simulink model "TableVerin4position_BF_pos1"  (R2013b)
settings: Solver=ode15s  StartTime=0.0  StopTime=10  RelTol=1e-3
undefined symbols (not defined in the file): deg, kg, m, mm, N, rad, s, X, Y, Z
libraries: sm_lib x907, fl_lib x24, nesl_utility x18, elec_lib x3, sdl_lib x2, simulink x1
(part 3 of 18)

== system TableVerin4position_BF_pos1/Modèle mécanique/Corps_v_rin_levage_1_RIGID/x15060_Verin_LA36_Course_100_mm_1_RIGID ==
  ReferenceFrame : sm_lib/Frames and Transforms/Reference Frame  BlockFunction=simmechanics.library.frames_transforms.reference_frame
  Solid : sm_lib/Body Elements/Solid  InertiaType=Custom  Mass=16.4344  MassUnits=kg  CenterOfMass=[-32.3232 0.0025488500000000001 17.760100000000001]  CenterOfMassUnits=mm  MomentsOfInertia=[90976.899999999994 107643 28123.599999999999]  MomentsOfInertiaUnits=kg*mm^2  ProductsOfInertia=[5.1204799999999997 -235.90300000000005 -1.9517]  ProductsOfInertiaUnits=kg*mm^2  DensityBased=on  Density=1000  DensityUnits=kg/(m^3)  GraphicType=FromGeometry  MarkerShape=Sphere  MarkerSize=10  MarkerSizeUnits=m  GraphicVisPropType=SimpleVisualProperties  GraphicDiffuseColor=[0.647059 0.517647 0]  GraphicSpecularColor=[0.5 0.5 0.5 1.0]  GraphicAmbientColor=[0.15 0.15 0.15 1.0]  GraphicEmissiveColor=[0.0 0.0 0.0 1.0]  GraphicShininess=75  GraphicOpacity=1  GeometryShape=FromFile  RectangleSize=[1 1]  RectangleSizeUnits=m  BrickDimensions=[1 1 1]  BrickDimensionUnits=m  CylinderRadius=1  CylinderRadiusUnits=m  CylinderLength=1  CylinderLengthUnits=m  SphereRadius=1  SphereRadiusUnits=m  EllipsoidRadii=[1 1 1]  EllipsoidRadiiUnits=m  ExtrusionCrossSection=[1 1; -1 1; -1 -1; 1 -1]  ExtrusionCrossSectionUnits=m  ExtrusionLength=1  ExtrusionLengthUnits=m  PolygonNumSides=3  PolygonOuterRadius=1  PolygonOuterRadiusUnits=m  ExtGeomFileName=15060-Verin - LA36 - Course 100 mm_Défaut_sldprt.STL  ExtGeomFileUnits=mm  RevolutionCrossSection=[1 1; 1 -1; 2 -1; 2 1]  RevolutionCrossSectionUnits=m  RevolutionExtent=Full  RevolutionAngle=180  RevolutionAngleUnits=deg  BlockFunction=simmechanics.library.body_elements.solid
  F : PMIOPort  Port=1  Side=Left
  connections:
  Solid/RConn1 -- ReferenceFrame/RConn1 -- F/RConn1

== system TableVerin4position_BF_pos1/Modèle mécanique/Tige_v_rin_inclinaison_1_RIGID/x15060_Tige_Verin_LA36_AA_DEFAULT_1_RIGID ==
  ReferenceFrame : sm_lib/Frames and Transforms/Reference Frame  BlockFunction=simmechanics.library.frames_transforms.reference_frame
  Solid : sm_lib/Body Elements/Solid  InertiaType=Custom  Mass=1.0865400000000001  MassUnits=kg  CenterOfMass=[100.095 0 0]  CenterOfMassUnits=mm  MomentsOfInertia=[122.032 3676.6300000000001 3676.6300000000001]  MomentsOfInertiaUnits=kg*mm^2  ProductsOfInertia=[0 0 0]  ProductsOfInertiaUnits=kg*mm^2  DensityBased=on  Density=1000  DensityUnits=kg/(m^3)  GraphicType=FromGeometry  MarkerShape=Sphere  MarkerSize=10  MarkerSizeUnits=m  GraphicVisPropType=SimpleVisualProperties  GraphicDiffuseColor=[0.776471 0.756863 0.737255]  GraphicSpecularColor=[0.5 0.5 0.5 1.0]  GraphicAmbientColor=[0.15 0.15 0.15 1.0]  GraphicEmissiveColor=[0.0 0.0 0.0 1.0]  GraphicShininess=75  GraphicOpacity=1  GeometryShape=FromFile  RectangleSize=[1 1]  RectangleSizeUnits=m  BrickDimensions=[1 1 1]  BrickDimensionUnits=m  CylinderRadius=1  CylinderRadiusUnits=m  CylinderLength=1  CylinderLengthUnits=m  SphereRadius=1  SphereRadiusUnits=m  EllipsoidRadii=[1 1 1]  EllipsoidRadiiUnits=m  ExtrusionCrossSection=[1 1; -1 1; -1 -1; 1 -1]  ExtrusionCrossSectionUnits=m  ExtrusionLength=1  ExtrusionLengthUnits=m  PolygonNumSides=3  PolygonOuterRadius=1  PolygonOuterRadiusUnits=m  ExtGeomFileName=15060-Tige Verin - LA36_AA - DEFAULT_Défaut_sldprt.STL  ExtGeomFileUnits=mm  RevolutionCrossSection=[1 1; 1 -1; 2 -1; 2 1]  RevolutionCrossSectionUnits=m  RevolutionExtent=Full  RevolutionAngle=180  RevolutionAngleUnits=deg  BlockFunction=simmechanics.library.body_elements.solid
  F : PMIOPort  Port=1  Side=Left
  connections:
  Solid/RConn1 -- ReferenceFrame/RConn1 -- F/RConn1

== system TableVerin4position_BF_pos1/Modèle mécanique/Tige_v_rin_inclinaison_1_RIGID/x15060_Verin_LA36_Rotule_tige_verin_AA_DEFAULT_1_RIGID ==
  ReferenceFrame : sm_lib/Frames and Transforms/Reference Frame  BlockFunction=simmechanics.library.frames_transforms.reference_frame
  Solid : sm_lib/Body Elements/Solid  InertiaType=Custom  Mass=0.218778  MassUnits=kg  CenterOfMass=[17.366699999999998 -1.65342e-06 4.7137100000000001e-06]  CenterOfMassUnits=mm  MomentsOfInertia=[24.659199999999998 72.896000000000001 84.362000000000009]  MomentsOfInertiaUnits=kg*mm^2  ProductsOfInertia=[-4.0241599999999998e-05 3.5702500000000002e-06 -2.8363700000000001e-06]  ProductsOfInertiaUnits=kg*mm^2  DensityBased=on  Density=1000  DensityUnits=kg/(m^3)  GraphicType=FromGeometry  MarkerShape=Sphere  MarkerSize=10  MarkerSizeUnits=m  GraphicVisPropType=SimpleVisualProperties  GraphicDiffuseColor=[0.776471 0.756863 0.737255]  GraphicSpecularColor=[0.5 0.5 0.5 1.0]  GraphicAmbientColor=[0.15 0.15 0.15 1.0]  GraphicEmissiveColor=[0.0 0.0 0.0 1.0]  GraphicShininess=75  GraphicOpacity=1  GeometryShape=FromFile  RectangleSize=[1 1]  RectangleSizeUnits=m  BrickDimensions=[1 1 1]  BrickDimensionUnits=m  CylinderRadius=1  CylinderRadiusUnits=m  CylinderLength=1  CylinderLengthUnits=m  SphereRadius=1  SphereRadiusUnits=m  EllipsoidRadii=[1 1 1]  EllipsoidRadiiUnits=m  ExtrusionCrossSection=[1 1; -1 1; -1 -1; 1 -1]  ExtrusionCrossSectionUnits=m  ExtrusionLength=1  ExtrusionLengthUnits=m  PolygonNumSides=3  PolygonOuterRadius=1  PolygonOuterRadiusUnits=m  ExtGeomFileName=15060-Verin - LA36 - Rotule tige verin_AA - DEFAULT_Défaut_sldprt.STL  ExtGeomFileUnits=mm  RevolutionCrossSection=[1 1; 1 -1; 2 -1; 2 1]  RevolutionCrossSectionUnits=m  RevolutionExtent=Full  RevolutionAngle=180  RevolutionAngleUnits=deg  BlockFunction=simmechanics.library.body_elements.solid
  F : PMIOPort  Port=1  Side=Left
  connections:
  Solid/RConn1 -- ReferenceFrame/RConn1 -- F/RConn1

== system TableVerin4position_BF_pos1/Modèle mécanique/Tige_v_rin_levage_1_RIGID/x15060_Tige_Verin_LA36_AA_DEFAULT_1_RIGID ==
  ReferenceFrame : sm_lib/Frames and Transforms/Reference Frame  BlockFunction=simmechanics.library.frames_transforms.reference_frame
  Solid : sm_lib/Body Elements/Solid  InertiaType=Custom  Mass=1.0865400000000001  MassUnits=kg  CenterOfMass=[100.095 0 0]  CenterOfMassUnits=mm  MomentsOfInertia=[122.032 3676.6300000000001 3676.6300000000001]  MomentsOfInertiaUnits=kg*mm^2  ProductsOfInertia=[0 0 0]  ProductsOfInertiaUnits=kg*mm^2  DensityBased=on  Density=1000  DensityUnits=kg/(m^3)  GraphicType=FromGeometry  MarkerShape=Sphere  MarkerSize=10  MarkerSizeUnits=m  GraphicVisPropType=SimpleVisualProperties  GraphicDiffuseColor=[0.776471 0.756863 0.737255]  GraphicSpecularColor=[0.5 0.5 0.5 1.0]  GraphicAmbientColor=[0.15 0.15 0.15 1.0]  GraphicEmissiveColor=[0.0 0.0 0.0 1.0]  GraphicShininess=75  GraphicOpacity=1  GeometryShape=FromFile  RectangleSize=[1 1]  RectangleSizeUnits=m  BrickDimensions=[1 1 1]  BrickDimensionUnits=m  CylinderRadius=1  CylinderRadiusUnits=m  CylinderLength=1  CylinderLengthUnits=m  SphereRadius=1  SphereRadiusUnits=m  EllipsoidRadii=[1 1 1]  EllipsoidRadiiUnits=m  ExtrusionCrossSection=[1 1; -1 1; -1 -1; 1 -1]  ExtrusionCrossSectionUnits=m  ExtrusionLength=1  ExtrusionLengthUnits=m  PolygonNumSides=3  PolygonOuterRadius=1  PolygonOuterRadiusUnits=m  ExtGeomFileName=15060-Tige Verin - LA36_AA - DEFAULT_Défaut_sldprt.STL  ExtGeomFileUnits=mm  RevolutionCrossSection=[1 1; 1 -1; 2 -1; 2 1]  RevolutionCrossSectionUnits=m  RevolutionExtent=Full  RevolutionAngle=180  RevolutionAngleUnits=deg  BlockFunction=simmechanics.library.body_elements.solid
  F : PMIOPort  Port=1  Side=Left
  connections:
  Solid/RConn1 -- ReferenceFrame/RConn1 -- F/RConn1

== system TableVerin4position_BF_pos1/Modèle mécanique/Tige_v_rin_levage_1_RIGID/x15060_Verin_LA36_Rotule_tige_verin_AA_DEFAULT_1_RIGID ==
  ReferenceFrame : sm_lib/Frames and Transforms/Reference Frame  BlockFunction=simmechanics.library.frames_transforms.reference_frame
  Solid : sm_lib/Body Elements/Solid  InertiaType=Custom  Mass=0.218778  MassUnits=kg  CenterOfMass=[17.366699999999998 -1.65342e-06 4.7137100000000001e-06]  CenterOfMassUnits=mm  MomentsOfInertia=[24.659199999999998 72.896000000000001 84.362000000000009]  MomentsOfInertiaUnits=kg*mm^2  ProductsOfInertia=[-4.0241599999999998e-05 3.5702500000000002e-06 -2.8363700000000001e-06]  ProductsOfInertiaUnits=kg*mm^2  DensityBased=on  Density=1000  DensityUnits=kg/(m^3)  GraphicType=FromGeometry  MarkerShape=Sphere  MarkerSize=10  MarkerSizeUnits=m  GraphicVisPropType=SimpleVisualProperties  GraphicDiffuseColor=[0.776471 0.756863 0.737255]  GraphicSpecularColor=[0.5 0.5 0.5 1.0]  GraphicAmbientColor=[0.15 0.15 0.15 1.0]  GraphicEmissiveColor=[0.0 0.0 0.0 1.0]  GraphicShininess=75  GraphicOpacity=1  GeometryShape=FromFile  RectangleSize=[1 1]  RectangleSizeUnits=m  BrickDimensions=[1 1 1]  BrickDimensionUnits=m  CylinderRadius=1  CylinderRadiusUnits=m  CylinderLength=1  CylinderLengthUnits=m  SphereRadius=1  SphereRadiusUnits=m  EllipsoidRadii=[1 1 1]  EllipsoidRadiiUnits=m  ExtrusionCrossSection=[1 1; -1 1; -1 -1; 1 -1]  ExtrusionCrossSectionUnits=m  ExtrusionLength=1  ExtrusionLengthUnits=m  PolygonNumSides=3  PolygonOuterRadius=1  PolygonOuterRadiusUnits=m  ExtGeomFileName=15060-Verin - LA36 - Rotule tige verin_AA - DEFAULT_Défaut_sldprt.STL  ExtGeomFileUnits=mm  RevolutionCrossSection=[1 1; 1 -1; 2 -1; 2 1]  RevolutionCrossSectionUnits=m  RevolutionExtent=Full  RevolutionAngle=180  RevolutionAngleUnits=deg  BlockFunction=simmechanics.library.body_elements.solid
  F : PMIOPort  Port=1  Side=Left
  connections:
  Solid/RConn1 -- ReferenceFrame/RConn1 -- F/RConn1

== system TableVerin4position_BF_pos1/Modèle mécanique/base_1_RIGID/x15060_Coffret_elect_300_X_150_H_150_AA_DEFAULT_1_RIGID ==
  ReferenceFrame : sm_lib/Frames and Transforms/Reference Frame  BlockFunction=simmechanics.library.frames_transforms.reference_frame
  Solid : sm_lib/Body Elements/Solid  InertiaType=Custom  Mass=0.83252499999999996  MassUnits=kg  CenterOfMass=[0 0 86.964399999999998]  CenterOfMassUnits=mm  MomentsOfInertia=[9125.25 3583.1799999999998 10424.799999999999]  MomentsOfInertiaUnits=kg*mm^2  ProductsOfInertia=[0 0 0]  ProductsOfInertiaUnits=kg*mm^2  DensityBased=on  Density=1000  DensityUnits=kg/(m^3)  GraphicType=FromGeometry  MarkerShape=Sphere  MarkerSize=10  MarkerSizeUnits=m  GraphicVisPropType=SimpleVisualProperties  GraphicDiffuseColor=[0.792157 0.819608 0.933333]  GraphicSpecularColor=[0.5 0.5 0.5 1.0]  GraphicAmbientColor=[0.15 0.15 0.15 1.0]  GraphicEmissiveColor=[0.0 0.0 0.0 1.0]  GraphicShininess=75  GraphicOpacity=1  GeometryShape=FromFile  RectangleSize=[1 1]  RectangleSizeUnits=m  BrickDimensions=[1 1 1]  BrickDimensionUnits=m  CylinderRadius=1  CylinderRadiusUnits=m  CylinderLength=1  CylinderLengthUnits=m  SphereRadius=1  SphereRadiusUnits=m  EllipsoidRadii=[1 1 1]  EllipsoidRadiiUnits=m  ExtrusionCrossSection=[1 1; -1 1; -1 -1; 1 -1]  ExtrusionCrossSectionUnits=m  ExtrusionLength=1  ExtrusionLengthUnits=m  PolygonNumSides=3  PolygonOuterRadius=1  PolygonOuterRadiusUnits=m  ExtGeomFileName=15060-Coffret elect - 300 X 150 H 150_AA - DEFAULT_Défaut_sldprt.STL  ExtGeomFileUnits=mm  RevolutionCrossSection=[1 1; 1 -1; 2 -1; 2 1]  RevolutionCrossSectionUnits=m  RevolutionExtent=Full  RevolutionAngle=180  RevolutionAngleUnits=deg  BlockFunction=simmechanics.library.body_elements.solid
  F : PMIOPort  Port=1  Side=Left
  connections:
  Solid/RConn1 -- ReferenceFrame/RConn1 -- F/RConn1

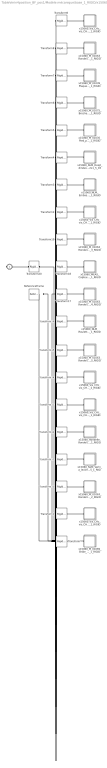
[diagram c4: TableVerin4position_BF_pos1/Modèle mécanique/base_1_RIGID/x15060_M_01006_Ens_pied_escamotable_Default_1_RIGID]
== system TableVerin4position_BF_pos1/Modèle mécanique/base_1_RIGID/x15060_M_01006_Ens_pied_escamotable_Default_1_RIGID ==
  ReferenceFrame : sm_lib/Frames and Transforms/Reference Frame  BlockFunction=simmechanics.library.frames_transforms.reference_frame
  Transform : sm_lib/Frames and Transforms/Rigid Transform  TranslationMethod=Cartesian  TranslationLengthUnit=mm  TranslationStandardAxis=+Z  TranslationStandardOffset=0  TranslationCartesianOffset=[-28 52.5 1]  TranslationROffset=0  TranslationROffsetUnits=m  TranslationZOffset=0  TranslationZOffsetUnits=m  TranslationThetaOffset=0  TranslationThetaOffsetUnits=deg  RotationMethod=ArbitraryAxis  RotationAngleUnits=rad  RotationStandardAxis=+Z  RotationAngle=2.0943951023931926  RotationArbitraryAxis=[-0.57735026918962484 0.57735026918962484 0.57735026918962762]  FollAlignAxisA=+X  BaseAlignAxisA=+Y  FollAlignAxisB=+Y  BaseAlignAxisB=+Z  BlockFunction=simmechanics.library.frames_transforms.rigid_transform
  Transform1 : sm_lib/Frames and Transforms/Rigid Transform  TranslationMethod=Cartesian  TranslationLengthUnit=mm  TranslationStandardAxis=+Z  TranslationStandardOffset=0  TranslationCartesianOffset=[-2 130 -15]  TranslationROffset=0  TranslationROffsetUnits=m  TranslationZOffset=0  TranslationZOffsetUnits=m  TranslationThetaOffset=0  TranslationThetaOffsetUnits=deg  RotationMethod=ArbitraryAxis  RotationAngleUnits=rad  RotationStandardAxis=+Z  RotationAngle=1.8468790707046723  RotationArbitraryAxis=[-0.46281772058563114 0.7560420061238935 -0.46281772058563114]  FollAlignAxisA=+X  BaseAlignAxisA=+Y  FollAlignAxisB=+Y  BaseAlignAxisB=+Z  BlockFunction=simmechanics.library.frames_transforms.rigid_transform
  Transform10 : sm_lib/Frames and Transforms/Rigid Transform  TranslationMethod=Cartesian  TranslationLengthUnit=mm  TranslationStandardAxis=+Z  TranslationStandardOffset=0  TranslationCartesianOffset=[-8 1 1]  TranslationROffset=0  TranslationROffsetUnits=m  TranslationZOffset=0  TranslationZOffsetUnits=m  TranslationThetaOffset=0  TranslationThetaOffsetUnits=deg  RotationMethod=ArbitraryAxis  RotationAngleUnits=rad  RotationStandardAxis=+Z  RotationAngle=2.5503618214833885  RotationArbitraryAxis=[0.67351920895470851 -0.6735192089547084 0.30453858595923028]  FollAlignAxisA=+X  BaseAlignAxisA=+Y  FollAlignAxisB=+Y  BaseAlignAxisB=+Z  BlockFunction=simmechanics.library.frames_transforms.rigid_transform
  Transform11 : sm_lib/Frames and Transforms/Rigid Transform  TranslationMethod=Cartesian  TranslationLengthUnit=mm  TranslationStandardAxis=+Z  TranslationStandardOffset=0  TranslationCartesianOffset=[-2 1 1]  TranslationROffset=0  TranslationROffsetUnits=m  TranslationZOffset=0  TranslationZOffsetUnits=m  TranslationThetaOffset=0  TranslationThetaOffsetUnits=deg  RotationMethod=ArbitraryAxis  RotationAngleUnits=rad  RotationStandardAxis=+Z  RotationAngle=0.78539829157538132  RotationArbitraryAxis=[-1 0 0]  FollAlignAxisA=+X  BaseAlignAxisA=+Y  FollAlignAxisB=+Y  BaseAlignAxisB=+Z  BlockFunction=simmechanics.library.frames_transforms.rigid_transform
  Transform12 : sm_lib/Frames and Transforms/Rigid Transform  TranslationMethod=Cartesian  TranslationLengthUnit=mm  TranslationStandardAxis=+Z  TranslationStandardOffset=0  TranslationCartesianOffset=[-69.299999999999997 1 1]  TranslationROffset=0  TranslationROffsetUnits=m  TranslationZOffset=0  TranslationZOffsetUnits=m  TranslationThetaOffset=0  TranslationThetaOffsetUnits=deg  RotationMethod=ArbitraryAxis  RotationAngleUnits=rad  RotationStandardAxis=+Z  RotationAngle=1.779666102874204  RotationArbitraryAxis=[-0.41441858134901061 -0.41441858134901077 -0.81025581075691555]  FollAlignAxisA=+X  BaseAlignAxisA=+Y  FollAlignAxisB=+Y  BaseAlignAxisB=+Z  BlockFunction=simmechanics.library.frames_transforms.rigid_transform
  Transform13 : sm_lib/Frames and Transforms/Rigid Transform  TranslationMethod=Cartesian  TranslationLengthUnit=mm  TranslationStandardAxis=+Z  TranslationStandardOffset=0  TranslationCartesianOffset=[23.5107 45 115]  TranslationROffset=0  TranslationROffsetUnits=m  TranslationZOffset=0  TranslationZOffsetUnits=m  TranslationThetaOffset=0  TranslationThetaOffsetUnits=deg  RotationMethod=ArbitraryAxis  RotationAngleUnits=rad  RotationStandardAxis=+Z  RotationAngle=1.7576864373908556  RotationArbitraryAxis=[0.39584132832668711 -0.82862493661313852 -0.39584132832668711]  FollAlignAxisA=+X  BaseAlignAxisA=+Y  FollAlignAxisB=+Y  BaseAlignAxisB=+Z  BlockFunction=simmechanics.library.frames_transforms.rigid_transform
  Transform14 : sm_lib/Frames and Transforms/Rigid Transform  TranslationMethod=Cartesian  TranslationLengthUnit=mm  TranslationStandardAxis=+Z  TranslationStandardOffset=0  TranslationCartesianOffset=[-2 -15 130]  TranslationROffset=0  TranslationROffsetUnits=m  TranslationZOffset=0  TranslationZOffsetUnits=m  TranslationThetaOffset=0  TranslationThetaOffsetUnits=deg  RotationMethod=ArbitraryAxis  RotationAngleUnits=rad  RotationStandardAxis=+Z  RotationAngle=1.8958525166545865  RotationArbitraryAxis=[-0.49199382426247901 0.7182507596760076 -0.49199382426247901]  FollAlignAxisA=+X  BaseAlignAxisA=+Y  FollAlignAxisB=+Y  BaseAlignAxisB=+Z  BlockFunction=simmechanics.library.frames_transforms.rigid_transform
  Transform15 : sm_lib/Frames and Transforms/Rigid Transform  TranslationMethod=Cartesian  TranslationLengthUnit=mm  TranslationStandardAxis=+Z  TranslationStandardOffset=0  TranslationCartesianOffset=[-7.0000000000000009 1 1]  TranslationROffset=0  TranslationROffsetUnits=m  TranslationZOffset=0  TranslationZOffsetUnits=m  TranslationThetaOffset=0  TranslationThetaOffsetUnits=deg  RotationMethod=ArbitraryAxis  RotationAngleUnits=rad  RotationStandardAxis=+Z  RotationAngle=2.5773215317098641  RotationArbitraryAxis=[0.6767483296554524 -0.67674832965545229 0.28986789511277461]  FollAlignAxisA=+X  BaseAlignAxisA=+Y  FollAlignAxisB=+Y  BaseAlignAxisB=+Z  BlockFunction=simmechanics.library.frames_transforms.rigid_transform
  Transform16 : sm_lib/Frames and Transforms/Rigid Transform  TranslationMethod=Cartesian  TranslationLengthUnit=mm  TranslationStandardAxis=+Z  TranslationStandardOffset=0  TranslationCartesianOffset=[73.5 50 85]  TranslationROffset=0  TranslationROffsetUnits=m  TranslationZOffset=0  TranslationZOffsetUnits=m  TranslationThetaOffset=0  TranslationThetaOffsetUnits=deg  RotationMethod=ArbitraryAxis  RotationAngleUnits=rad  RotationStandardAxis=+Z  RotationAngle=1.5707963267948968  RotationArbitraryAxis=[0 0 1]  FollAlignAxisA=+X  BaseAlignAxisA=+Y  FollAlignAxisB=+Y  BaseAlignAxisB=+Z  BlockFunction=simmechanics.library.frames_transforms.rigid_transform
  Transform17 : sm_lib/Frames and Transforms/Rigid Transform  TranslationMethod=Cartesian  TranslationLengthUnit=mm  TranslationStandardAxis=+Z  TranslationStandardOffset=0  TranslationCartesianOffset=[-9 1 1]  TranslationROffset=0  TranslationROffsetUnits=m  TranslationZOffset=0  TranslationZOffsetUnits=m  TranslationThetaOffset=0  TranslationThetaOffsetUnits=deg  RotationMethod=ArbitraryAxis  RotationAngleUnits=rad  RotationStandardAxis=+Z  RotationAngle=2.5503618214833885  RotationArbitraryAxis=[0.67351920895470851 -0.6735192089547084 0.30453858595923028]  FollAlignAxisA=+X  BaseAlignAxisA=+Y  FollAlignAxisB=+Y  BaseAlignAxisB=+Z  BlockFunction=simmechanics.library.frames_transforms.rigid_transform
  Transform18 : sm_lib/Frames and Transforms/Rigid Transform  TranslationMethod=Cartesian  TranslationLengthUnit=mm  TranslationStandardAxis=+Z  TranslationStandardOffset=0  TranslationCartesianOffset=[14 1 1]  TranslationROffset=0  TranslationROffsetUnits=m  TranslationZOffset=0  TranslationZOffsetUnits=m  TranslationThetaOffset=0  TranslationThetaOffsetUnits=deg  RotationMethod=ArbitraryAxis  RotationAngleUnits=rad  RotationStandardAxis=+Z  RotationAngle=2.0943951023931953  RotationArbitraryAxis=[-0.57735026918962584 0.57735026918962584 0.57735026918962584]  FollAlignAxisA=+X  BaseAlignAxisA=+Y  FollAlignAxisB=+Y  BaseAlignAxisB=+Z  BlockFunction=simmechanics.library.frames_transforms.rigid_transform
  Transform19 : sm_lib/Frames and Transforms/Rigid Transform  TranslationMethod=Cartesian  TranslationLengthUnit=mm  TranslationStandardAxis=+Z  TranslationStandardOffset=0  TranslationCartesianOffset=[-6 1 1]  TranslationROffset=0  TranslationROffsetUnits=m  TranslationZOffset=0  TranslationZOffsetUnits=m  TranslationThetaOffset=0  TranslationThetaOffsetUnits=deg  RotationMethod=ArbitraryAxis  RotationAngleUnits=rad  RotationStandardAxis=+Z  RotationAngle=2.5773215317098641  RotationArbitraryAxis=[0.6767483296554524 -0.6767483296554524 0.28986789511277455]  FollAlignAxisA=+X  BaseAlignAxisA=+Y  FollAlignAxisB=+Y  BaseAlignAxisB=+Z  BlockFunction=simmechanics.library.frames_transforms.rigid_transform
  Transform2 : sm_lib/Frames and Transforms/Rigid Transform  TranslationMethod=Cartesian  TranslationLengthUnit=mm  TranslationStandardAxis=+Z  TranslationStandardOffset=0  TranslationCartesianOffset=[-75.300000000000011 1 1]  TranslationROffset=0  TranslationROffsetUnits=m  TranslationZOffset=0  TranslationZOffsetUnits=m  TranslationThetaOffset=0  TranslationThetaOffsetUnits=deg  RotationMethod=ArbitraryAxis  RotationAngleUnits=rad  RotationStandardAxis=+Z  RotationAngle=2.533359793208557  RotationArbitraryAxis=[-0.67137794896695524 0.31385235267853073 -0.67137794896695535]  FollAlignAxisA=+X  BaseAlignAxisA=+Y  FollAlignAxisB=+Y  BaseAlignAxisB=+Z  BlockFunction=simmechanics.library.frames_transforms.rigid_transform
  Transform20 : sm_lib/Frames and Transforms/Rigid Transform  TranslationMethod=Cartesian  TranslationLengthUnit=mm  TranslationStandardAxis=+Z  TranslationStandardOffset=0  TranslationCartesianOffset=[-1705 -380 33]  TranslationROffset=0  TranslationROffsetUnits=m  TranslationZOffset=0  TranslationZOffsetUnits=m  TranslationThetaOffset=0  TranslationThetaOffsetUnits=deg  RotationMethod=ArbitraryAxis  RotationAngleUnits=rad  RotationStandardAxis=+Z  RotationAngle=1.5707963267948939  RotationArbitraryAxis=[1.6938670000000002e-15 1 9.0283299999999997e-16]  FollAlignAxisA=+X  BaseAlignAxisA=+Y  FollAlignAxisB=+Y  BaseAlignAxisB=+Z  BlockFunction=simmechanics.library.frames_transforms.rigid_transform
  Transform3 : sm_lib/Frames and Transforms/Rigid Transform  TranslationMethod=Cartesian  TranslationLengthUnit=mm  TranslationStandardAxis=+Z  TranslationStandardOffset=0  TranslationCartesianOffset=[104 1 1]  TranslationROffset=0  TranslationROffsetUnits=m  TranslationZOffset=0  TranslationZOffsetUnits=m  TranslationThetaOffset=0  TranslationThetaOffsetUnits=deg  RotationMethod=ArbitraryAxis  RotationAngleUnits=rad  RotationStandardAxis=+Z  RotationAngle=2.8467308529659632  RotationArbitraryAxis=[-0.6992657722290897 0.6992657722290897 0.14850844951621375]  FollAlignAxisA=+X  BaseAlignAxisA=+Y  FollAlignAxisB=+Y  BaseAlignAxisB=+Z  BlockFunction=simmechanics.library.frames_transforms.rigid_transform
  Transform4 : sm_lib/Frames and Transforms/Rigid Transform  TranslationMethod=Cartesian  TranslationLengthUnit=mm  TranslationStandardAxis=+Z  TranslationStandardOffset=0  TranslationCartesianOffset=[-3 52.5 -23]  TranslationROffset=0  TranslationROffsetUnits=m  TranslationZOffset=0  TranslationZOffsetUnits=m  TranslationThetaOffset=0  TranslationThetaOffsetUnits=deg  RotationMethod=ArbitraryAxis  RotationAngleUnits=rad  RotationStandardAxis=+Z  RotationAngle=1.6378338521091518  RotationArbitraryAxis=[-0.25056285449650229 0.25056285449650229 0.9351131011236713]  FollAlignAxisA=+X  BaseAlignAxisA=+Y  FollAlignAxisB=+Y  BaseAlignAxisB=+Z  BlockFunction=simmechanics.library.frames_transforms.rigid_transform
  Transform5 : sm_lib/Frames and Transforms/Rigid Transform  TranslationMethod=Cartesian  TranslationLengthUnit=mm  TranslationStandardAxis=+Z  TranslationStandardOffset=0  TranslationCartesianOffset=[26 1 1]  TranslationROffset=0  TranslationROffsetUnits=m  TranslationZOffset=0  TranslationZOffsetUnits=m  TranslationThetaOffset=0  TranslationThetaOffsetUnits=deg  RotationMethod=ArbitraryAxis  RotationAngleUnits=rad  RotationStandardAxis=+Z  RotationAngle=1.5964112029521187  RotationArbitraryAxis=[-0.15802682740811666 0.15802682740811666 0.97470767086273136]  FollAlignAxisA=+X  BaseAlignAxisA=+Y  FollAlignAxisB=+Y  BaseAlignAxisB=+Z  BlockFunction=simmechanics.library.frames_transforms.rigid_transform
  Transform6 : sm_lib/Frames and Transforms/Rigid Transform  TranslationMethod=Cartesian  TranslationLengthUnit=mm  TranslationStandardAxis=+Z  TranslationStandardOffset=0  TranslationCartesianOffset=[74 1 1]  TranslationROffset=0  TranslationROffsetUnits=m  TranslationZOffset=0  TranslationZOffsetUnits=m  TranslationThetaOffset=0  TranslationThetaOffsetUnits=deg  RotationMethod=ArbitraryAxis  RotationAngleUnits=rad  RotationStandardAxis=+Z  RotationAngle=3.1415926535897931  RotationArbitraryAxis=[3.1925426677448238e-17 0.91204751904576642 0.41008453153278329]  FollAlignAxisA=+X  BaseAlignAxisA=+Y  FollAlignAxisB=+Y  BaseAlignAxisB=+Z  BlockFunction=simmechanics.library.frames_transforms.rigid_transform
  Transform7 : sm_lib/Frames and Transforms/Rigid Transform  TranslationMethod=Cartesian  TranslationLengthUnit=mm  TranslationStandardAxis=+Z  TranslationStandardOffset=0  TranslationCartesianOffset=[13 85 85]  TranslationROffset=0  TranslationROffsetUnits=m  TranslationZOffset=0  TranslationZOffsetUnits=m  TranslationThetaOffset=0  TranslationThetaOffsetUnits=deg  RotationMethod=ArbitraryAxis  RotationAngleUnits=rad  RotationStandardAxis=+Z  RotationAngle=1.5707963267948939  RotationArbitraryAxis=[-1.6938670000000002e-15 -1 -9.0283299999999997e-16]  FollAlignAxisA=+X  BaseAlignAxisA=+Y  FollAlignAxisB=+Y  BaseAlignAxisB=+Z  BlockFunction=simmechanics.library.frames_transforms.rigid_transform
  Transform8 : sm_lib/Frames and Transforms/Rigid Transform  TranslationMethod=Cartesian  TranslationLengthUnit=mm  TranslationStandardAxis=+Z  TranslationStandardOffset=0  TranslationCartesianOffset=[-10 1 1]  TranslationROffset=0  TranslationROffsetUnits=m  TranslationZOffset=0  TranslationZOffsetUnits=m  TranslationThetaOffset=0  TranslationThetaOffsetUnits=deg  RotationMethod=ArbitraryAxis  RotationAngleUnits=rad  RotationStandardAxis=+Z  RotationAngle=2.5503618214833885  RotationArbitraryAxis=[0.67351920895470851 -0.6735192089547084 0.30453858595923028]  FollAlignAxisA=+X  BaseAlignAxisA=+Y  FollAlignAxisB=+Y  BaseAlignAxisB=+Z  BlockFunction=simmechanics.library.frames_transforms.rigid_transform
  Transform9 : sm_lib/Frames and Transforms/Rigid Transform  TranslationMethod=Cartesian  TranslationLengthUnit=mm  TranslationStandardAxis=+Z  TranslationStandardOffset=0  TranslationCartesianOffset=[-39 52.5 19]  TranslationROffset=0  TranslationROffsetUnits=m  TranslationZOffset=0  TranslationZOffsetUnits=m  TranslationThetaOffset=0  TranslationThetaOffsetUnits=deg  RotationMethod=ArbitraryAxis  RotationAngleUnits=rad  RotationStandardAxis=+Z  RotationAngle=3.1415926535897905  RotationArbitraryAxis=[-0.57504174666649199 0.81812406735821563 2.040515663386459e-15]  FollAlignAxisA=+X  BaseAlignAxisA=+Y  FollAlignAxisB=+Y  BaseAlignAxisB=+Z  BlockFunction=simmechanics.library.frames_transforms.rigid_transform
  x15060_MEAS_Capteur_deffort_1000_N_FN_9620_AA_DEFAULT_1_RIGID : Subsystem
  x15060_M_01035_Pied_porte_capteur_AA_DEFAULT_1_RIGID : Subsystem
  x15060_M_01039_Plaque_roulette_AA_DEFAULT_1_RIGID : Subsystem
  x15060_M_01063_Rondelle_entretoise_AA_DEFAULT_1_RIGID : Subsystem
  x15060_M_01063_Rondelle_entretoise_AA_DEFAULT_2_RIGID : Subsystem
  x15060_M_01063_Rondelle_entretoise_AA_DEFAULT_3_RIGID : Subsystem
  x15060_M_01063_Rondelle_entretoise_AA_DEFAULT_4_RIGID : Subsystem
  x15060_M_01063_Rondelle_entretoise_AA_DEFAULT_5_RIGID : Subsystem
  x15060_M_01069_Bride_doigt_dindexage_AA_DEFAULT_1_RIGID : Subsystem
  x15060_M_01075_Broche_M12_Modifi_e_27810_120451_1_RIGID : Subsystem
  x15060_NLM_Doigt_dindexage_acier_6_avec_contre_ecrou_M12x1_5_03 : Subsystem
  x15060_NLM_Embase_60_27801_20601_1_RIGID : Subsystem
  x15060_NLM_Roulette_pivotante_F_200_KG_95034_07532_1_RIGID : Subsystem
  x15060_NLM_Verin_a_levier_Rot_a_droite_traction_04410_35_1_RIGI : Subsystem
  x15060_Rondelle_Rondelle_Large_L_6_1_RIGID : Subsystem
  x15060_Vis_CHc_vis_CHc_M_5_X_20_1_RIGID : Subsystem
  x15060_Vis_CHc_vis_CHc_M_6_X_16_1_RIGID : Subsystem
  x15060_Vis_CHc_vis_CHc_M_8_X_12_1_RIGID : Subsystem
  x15060_Vis_CHc_vis_CHc_M_8_X_25_1_RIGID : Subsystem
  x15060_Vis_CHc_vis_CHc_M_8_X_25_2_RIGID : Subsystem
  F : PMIOPort  Port=1  Side=Right
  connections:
  Transform/RConn1 -- x15060_M_01069_Bride_doigt_dindexage_AA_DEFAULT_1_RIGID/LConn1
  Transform1/RConn1 -- x15060_Vis_CHc_vis_CHc_M_8_X_25_1_RIGID/LConn1
  Transform10/RConn1 -- x15060_M_01063_Rondelle_entretoise_AA_DEFAULT_2_RIGID/LConn1
  Transform11/RConn1 -- x15060_NLM_Verin_a_levier_Rot_a_droite_traction_04410_35_1_RIGI/LConn1
  Transform12/RConn1 -- x15060_Rondelle_Rondelle_Large_L_6_1_RIGID/LConn1
  Transform13/RConn1 -- x15060_Vis_CHc_vis_CHc_M_8_X_12_1_RIGID/LConn1
  Transform14/RConn1 -- x15060_Vis_CHc_vis_CHc_M_8_X_25_2_RIGID/LConn1
  Transform15/RConn1 -- x15060_M_01063_Rondelle_entretoise_AA_DEFAULT_5_RIGID/LConn1
  Transform16/RConn1 -- x15060_NLM_Roulette_pivotante_F_200_KG_95034_07532_1_RIGID/LConn1
  Transform17/RConn1 -- x15060_M_01063_Rondelle_entretoise_AA_DEFAULT_4_RIGID/LConn1
  Transform18/RConn1 -- x15060_MEAS_Capteur_deffort_1000_N_FN_9620_AA_DEFAULT_1_RIGID/LConn1
  Transform19/RConn1 -- x15060_M_01063_Rondelle_entretoise_AA_DEFAULT_3_RIGID/LConn1
  Transform2/RConn1 -- x15060_Vis_CHc_vis_CHc_M_6_X_16_1_RIGID/LConn1
  Transform/LConn1 -- ReferenceFrame/RConn1 -- Transform1/LConn1 -- Transform10/LConn1 -- Transform11/LConn1 -- Transform12/LConn1 -- Transform13/LConn1 -- Transform14/LConn1 -- Transform15/LConn1 -- Transform16/LConn1 -- Transform17/LConn1 -- Transform18/LConn1 -- Transform19/LConn1 -- Transform2/LConn1 -- Transform20/RConn1 -- Transform3/LConn1 -- Transform4/LConn1 -- Transform5/LConn1 -- Transform6/LConn1 -- Transform7/LConn1 -- Transform8/LConn1 -- Transform9/LConn1
  Transform20/LConn1 -- F/RConn1
  Transform3/RConn1 -- x15060_NLM_Embase_60_27801_20601_1_RIGID/LConn1
  Transform4/RConn1 -- x15060_NLM_Doigt_dindexage_acier_6_avec_contre_ecrou_M12x1_5_03/LConn1
  Transform5/RConn1 -- x15060_M_01035_Pied_porte_capteur_AA_DEFAULT_1_RIGID/LConn1
  Transform6/RConn1 -- x15060_M_01075_Broche_M12_Modifi_e_27810_120451_1_RIGID/LConn1
  Transform7/RConn1 -- x15060_M_01039_Plaque_roulette_AA_DEFAULT_1_RIGID/LConn1
  Transform8/RConn1 -- x15060_M_01063_Rondelle_entretoise_AA_DEFAULT_1_RIGID/LConn1
  Transform9/RConn1 -- x15060_Vis_CHc_vis_CHc_M_5_X_20_1_RIGID/LConn1

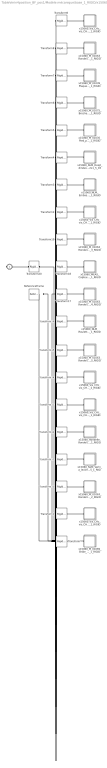
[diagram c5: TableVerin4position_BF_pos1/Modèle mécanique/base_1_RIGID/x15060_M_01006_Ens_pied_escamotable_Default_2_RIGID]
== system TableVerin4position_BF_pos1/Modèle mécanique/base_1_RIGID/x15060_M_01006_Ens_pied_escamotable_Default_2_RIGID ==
  ReferenceFrame : sm_lib/Frames and Transforms/Reference Frame  BlockFunction=simmechanics.library.frames_transforms.reference_frame
  Transform : sm_lib/Frames and Transforms/Rigid Transform  TranslationMethod=Cartesian  TranslationLengthUnit=mm  TranslationStandardAxis=+Z  TranslationStandardOffset=0  TranslationCartesianOffset=[-28 52.5 1]  TranslationROffset=0  TranslationROffsetUnits=m  TranslationZOffset=0  TranslationZOffsetUnits=m  TranslationThetaOffset=0  TranslationThetaOffsetUnits=deg  RotationMethod=ArbitraryAxis  RotationAngleUnits=rad  RotationStandardAxis=+Z  RotationAngle=2.0943951023931926  RotationArbitraryAxis=[-0.57735026918962484 0.57735026918962484 0.57735026918962762]  FollAlignAxisA=+X  BaseAlignAxisA=+Y  FollAlignAxisB=+Y  BaseAlignAxisB=+Z  BlockFunction=simmechanics.library.frames_transforms.rigid_transform
  Transform1 : sm_lib/Frames and Transforms/Rigid Transform  TranslationMethod=Cartesian  TranslationLengthUnit=mm  TranslationStandardAxis=+Z  TranslationStandardOffset=0  TranslationCartesianOffset=[-2 130 -15]  TranslationROffset=0  TranslationROffsetUnits=m  TranslationZOffset=0  TranslationZOffsetUnits=m  TranslationThetaOffset=0  TranslationThetaOffsetUnits=deg  RotationMethod=ArbitraryAxis  RotationAngleUnits=rad  RotationStandardAxis=+Z  RotationAngle=1.8468790707046723  RotationArbitraryAxis=[-0.46281772058563114 0.7560420061238935 -0.46281772058563114]  FollAlignAxisA=+X  BaseAlignAxisA=+Y  FollAlignAxisB=+Y  BaseAlignAxisB=+Z  BlockFunction=simmechanics.library.frames_transforms.rigid_transform
  Transform10 : sm_lib/Frames and Transforms/Rigid Transform  TranslationMethod=Cartesian  TranslationLengthUnit=mm  TranslationStandardAxis=+Z  TranslationStandardOffset=0  TranslationCartesianOffset=[-8 1 1]  TranslationROffset=0  TranslationROffsetUnits=m  TranslationZOffset=0  TranslationZOffsetUnits=m  TranslationThetaOffset=0  TranslationThetaOffsetUnits=deg  RotationMethod=ArbitraryAxis  RotationAngleUnits=rad  RotationStandardAxis=+Z  RotationAngle=2.5503618214833885  RotationArbitraryAxis=[0.67351920895470851 -0.6735192089547084 0.30453858595923028]  FollAlignAxisA=+X  BaseAlignAxisA=+Y  FollAlignAxisB=+Y  BaseAlignAxisB=+Z  BlockFunction=simmechanics.library.frames_transforms.rigid_transform
  Transform11 : sm_lib/Frames and Transforms/Rigid Transform  TranslationMethod=Cartesian  TranslationLengthUnit=mm  TranslationStandardAxis=+Z  TranslationStandardOffset=0  TranslationCartesianOffset=[-2 1 1]  TranslationROffset=0  TranslationROffsetUnits=m  TranslationZOffset=0  TranslationZOffsetUnits=m  TranslationThetaOffset=0  TranslationThetaOffsetUnits=deg  RotationMethod=ArbitraryAxis  RotationAngleUnits=rad  RotationStandardAxis=+Z  RotationAngle=0.78539829157538132  RotationArbitraryAxis=[-1 0 0]  FollAlignAxisA=+X  BaseAlignAxisA=+Y  FollAlignAxisB=+Y  BaseAlignAxisB=+Z  BlockFunction=simmechanics.library.frames_transforms.rigid_transform
  Transform12 : sm_lib/Frames and Transforms/Rigid Transform  TranslationMethod=Cartesian  TranslationLengthUnit=mm  TranslationStandardAxis=+Z  TranslationStandardOffset=0  TranslationCartesianOffset=[-69.299999999999997 1 1]  TranslationROffset=0  TranslationROffsetUnits=m  TranslationZOffset=0  TranslationZOffsetUnits=m  TranslationThetaOffset=0  TranslationThetaOffsetUnits=deg  RotationMethod=ArbitraryAxis  RotationAngleUnits=rad  RotationStandardAxis=+Z  RotationAngle=1.779666102874204  RotationArbitraryAxis=[-0.41441858134901061 -0.41441858134901077 -0.81025581075691555]  FollAlignAxisA=+X  BaseAlignAxisA=+Y  FollAlignAxisB=+Y  BaseAlignAxisB=+Z  BlockFunction=simmechanics.library.frames_transforms.rigid_transform
  Transform13 : sm_lib/Frames and Transforms/Rigid Transform  TranslationMethod=Cartesian  TranslationLengthUnit=mm  TranslationStandardAxis=+Z  TranslationStandardOffset=0  TranslationCartesianOffset=[23.5107 45 115]  TranslationROffset=0  TranslationROffsetUnits=m  TranslationZOffset=0  TranslationZOffsetUnits=m  TranslationThetaOffset=0  TranslationThetaOffsetUnits=deg  RotationMethod=ArbitraryAxis  RotationAngleUnits=rad  RotationStandardAxis=+Z  RotationAngle=1.7576864373908556  RotationArbitraryAxis=[0.39584132832668711 -0.82862493661313852 -0.39584132832668711]  FollAlignAxisA=+X  BaseAlignAxisA=+Y  FollAlignAxisB=+Y  BaseAlignAxisB=+Z  BlockFunction=simmechanics.library.frames_transforms.rigid_transform
  Transform14 : sm_lib/Frames and Transforms/Rigid Transform  TranslationMethod=Cartesian  TranslationLengthUnit=mm  TranslationStandardAxis=+Z  TranslationStandardOffset=0  TranslationCartesianOffset=[-2 -15 130]  TranslationROffset=0  TranslationROffsetUnits=m  TranslationZOffset=0  TranslationZOffsetUnits=m  TranslationThetaOffset=0  TranslationThetaOffsetUnits=deg  RotationMethod=ArbitraryAxis  RotationAngleUnits=rad  RotationStandardAxis=+Z  RotationAngle=1.8958525166545865  RotationArbitraryAxis=[-0.49199382426247901 0.7182507596760076 -0.49199382426247901]  FollAlignAxisA=+X  BaseAlignAxisA=+Y  FollAlignAxisB=+Y  BaseAlignAxisB=+Z  BlockFunction=simmechanics.library.frames_transforms.rigid_transform
  Transform15 : sm_lib/Frames and Transforms/Rigid Transform  TranslationMethod=Cartesian  TranslationLengthUnit=mm  TranslationStandardAxis=+Z  TranslationStandardOffset=0  TranslationCartesianOffset=[-7.0000000000000009 1 1]  TranslationROffset=0  TranslationROffsetUnits=m  TranslationZOffset=0  TranslationZOffsetUnits=m  TranslationThetaOffset=0  TranslationThetaOffsetUnits=deg  RotationMethod=ArbitraryAxis  RotationAngleUnits=rad  RotationStandardAxis=+Z  RotationAngle=2.5773215317098641  RotationArbitraryAxis=[0.6767483296554524 -0.67674832965545229 0.28986789511277461]  FollAlignAxisA=+X  BaseAlignAxisA=+Y  FollAlignAxisB=+Y  BaseAlignAxisB=+Z  BlockFunction=simmechanics.library.frames_transforms.rigid_transform
  Transform16 : sm_lib/Frames and Transforms/Rigid Transform  TranslationMethod=Cartesian  TranslationLengthUnit=mm  TranslationStandardAxis=+Z  TranslationStandardOffset=0  TranslationCartesianOffset=[73.5 50 85]  TranslationROffset=0  TranslationROffsetUnits=m  TranslationZOffset=0  TranslationZOffsetUnits=m  TranslationThetaOffset=0  TranslationThetaOffsetUnits=deg  RotationMethod=ArbitraryAxis  RotationAngleUnits=rad  RotationStandardAxis=+Z  RotationAngle=1.5707963267948968  RotationArbitraryAxis=[0 0 1]  FollAlignAxisA=+X  BaseAlignAxisA=+Y  FollAlignAxisB=+Y  BaseAlignAxisB=+Z  BlockFunction=simmechanics.library.frames_transforms.rigid_transform
  Transform17 : sm_lib/Frames and Transforms/Rigid Transform  TranslationMethod=Cartesian  TranslationLengthUnit=mm  TranslationStandardAxis=+Z  TranslationStandardOffset=0  TranslationCartesianOffset=[-9 1 1]  TranslationROffset=0  TranslationROffsetUnits=m  TranslationZOffset=0  TranslationZOffsetUnits=m  TranslationThetaOffset=0  TranslationThetaOffsetUnits=deg  RotationMethod=ArbitraryAxis  RotationAngleUnits=rad  RotationStandardAxis=+Z  RotationAngle=2.5503618214833885  RotationArbitraryAxis=[0.67351920895470851 -0.6735192089547084 0.30453858595923028]  FollAlignAxisA=+X  BaseAlignAxisA=+Y  FollAlignAxisB=+Y  BaseAlignAxisB=+Z  BlockFunction=simmechanics.library.frames_transforms.rigid_transform
  Transform18 : sm_lib/Frames and Transforms/Rigid Transform  TranslationMethod=Cartesian  TranslationLengthUnit=mm  TranslationStandardAxis=+Z  TranslationStandardOffset=0  TranslationCartesianOffset=[14 1 1]  TranslationROffset=0  TranslationROffsetUnits=m  TranslationZOffset=0  TranslationZOffsetUnits=m  TranslationThetaOffset=0  TranslationThetaOffsetUnits=deg  RotationMethod=ArbitraryAxis  RotationAngleUnits=rad  RotationStandardAxis=+Z  RotationAngle=2.0943951023931953  RotationArbitraryAxis=[-0.57735026918962584 0.57735026918962584 0.57735026918962584]  FollAlignAxisA=+X  BaseAlignAxisA=+Y  FollAlignAxisB=+Y  BaseAlignAxisB=+Z  BlockFunction=simmechanics.library.frames_transforms.rigid_transform
  Transform19 : sm_lib/Frames and Transforms/Rigid Transform  TranslationMethod=Cartesian  TranslationLengthUnit=mm  TranslationStandardAxis=+Z  TranslationStandardOffset=0  TranslationCartesianOffset=[-6 1 1]  TranslationROffset=0  TranslationROffsetUnits=m  TranslationZOffset=0  TranslationZOffsetUnits=m  TranslationThetaOffset=0  TranslationThetaOffsetUnits=deg  RotationMethod=ArbitraryAxis  RotationAngleUnits=rad  RotationStandardAxis=+Z  RotationAngle=2.5773215317098641  RotationArbitraryAxis=[0.6767483296554524 -0.6767483296554524 0.28986789511277455]  FollAlignAxisA=+X  BaseAlignAxisA=+Y  FollAlignAxisB=+Y  BaseAlignAxisB=+Z  BlockFunction=simmechanics.library.frames_transforms.rigid_transform
  Transform2 : sm_lib/Frames and Transforms/Rigid Transform  TranslationMethod=Cartesian  TranslationLengthUnit=mm  TranslationStandardAxis=+Z  TranslationStandardOffset=0  TranslationCartesianOffset=[-75.300000000000011 1 1]  TranslationROffset=0  TranslationROffsetUnits=m  TranslationZOffset=0  TranslationZOffsetUnits=m  TranslationThetaOffset=0  TranslationThetaOffsetUnits=deg  RotationMethod=ArbitraryAxis  RotationAngleUnits=rad  RotationStandardAxis=+Z  RotationAngle=2.533359793208557  RotationArbitraryAxis=[-0.67137794896695524 0.31385235267853073 -0.67137794896695535]  FollAlignAxisA=+X  BaseAlignAxisA=+Y  FollAlignAxisB=+Y  BaseAlignAxisB=+Z  BlockFunction=simmechanics.library.frames_transforms.rigid_transform
  Transform20 : sm_lib/Frames and Transforms/Rigid Transform  TranslationMethod=Cartesian  TranslationLengthUnit=mm  TranslationStandardAxis=+Z  TranslationStandardOffset=0  TranslationCartesianOffset=[-1705 380 33]  TranslationROffset=0  TranslationROffsetUnits=m  TranslationZOffset=0  TranslationZOffsetUnits=m  TranslationThetaOffset=0  TranslationThetaOffsetUnits=deg  RotationMethod=ArbitraryAxis  RotationAngleUnits=rad  RotationStandardAxis=+Z  RotationAngle=2.0943951023931957  RotationArbitraryAxis=[0.5773502691896274 0.57735026918962562 -0.57735026918962429]  FollAlignAxisA=+X  BaseAlignAxisA=+Y  FollAlignAxisB=+Y  BaseAlignAxisB=+Z  BlockFunction=simmechanics.library.frames_transforms.rigid_transform
  Transform3 : sm_lib/Frames and Transforms/Rigid Transform  TranslationMethod=Cartesian  TranslationLengthUnit=mm  TranslationStandardAxis=+Z  TranslationStandardOffset=0  TranslationCartesianOffset=[104 1 1]  TranslationROffset=0  TranslationROffsetUnits=m  TranslationZOffset=0  TranslationZOffsetUnits=m  TranslationThetaOffset=0  TranslationThetaOffsetUnits=deg  RotationMethod=ArbitraryAxis  RotationAngleUnits=rad  RotationStandardAxis=+Z  RotationAngle=2.8467308529659632  RotationArbitraryAxis=[-0.6992657722290897 0.6992657722290897 0.14850844951621375]  FollAlignAxisA=+X  BaseAlignAxisA=+Y  FollAlignAxisB=+Y  BaseAlignAxisB=+Z  BlockFunction=simmechanics.library.frames_transforms.rigid_transform
  Transform4 : sm_lib/Frames and Transforms/Rigid Transform  TranslationMethod=Cartesian  TranslationLengthUnit=mm  TranslationStandardAxis=+Z  TranslationStandardOffset=0  TranslationCartesianOffset=[-3 52.5 -23]  TranslationROffset=0  TranslationROffsetUnits=m  TranslationZOffset=0  TranslationZOffsetUnits=m  TranslationThetaOffset=0  TranslationThetaOffsetUnits=deg  RotationMethod=ArbitraryAxis  RotationAngleUnits=rad  RotationStandardAxis=+Z  RotationAngle=1.6378338521091518  RotationArbitraryAxis=[-0.25056285449650229 0.25056285449650229 0.9351131011236713]  FollAlignAxisA=+X  BaseAlignAxisA=+Y  FollAlignAxisB=+Y  BaseAlignAxisB=+Z  BlockFunction=simmechanics.library.frames_transforms.rigid_transform
  Transform5 : sm_lib/Frames and Transforms/Rigid Transform  TranslationMethod=Cartesian  TranslationLengthUnit=mm  TranslationStandardAxis=+Z  TranslationStandardOffset=0  TranslationCartesianOffset=[26 1 1]  TranslationROffset=0  TranslationROffsetUnits=m  TranslationZOffset=0  TranslationZOffsetUnits=m  TranslationThetaOffset=0  TranslationThetaOffsetUnits=deg  RotationMethod=ArbitraryAxis  RotationAngleUnits=rad  RotationStandardAxis=+Z  RotationAngle=1.5964112029521187  RotationArbitraryAxis=[-0.15802682740811666 0.15802682740811666 0.97470767086273136]  FollAlignAxisA=+X  BaseAlignAxisA=+Y  FollAlignAxisB=+Y  BaseAlignAxisB=+Z  BlockFunction=simmechanics.library.frames_transforms.rigid_transform
  Transform6 : sm_lib/Frames and Transforms/Rigid Transform  TranslationMethod=Cartesian  TranslationLengthUnit=mm  TranslationStandardAxis=+Z  TranslationStandardOffset=0  TranslationCartesianOffset=[74 1 1]  TranslationROffset=0  TranslationROffsetUnits=m  TranslationZOffset=0  TranslationZOffsetUnits=m  TranslationThetaOffset=0  TranslationThetaOffsetUnits=deg  RotationMethod=ArbitraryAxis  RotationAngleUnits=rad  RotationStandardAxis=+Z  RotationAngle=3.1415926535897931  RotationArbitraryAxis=[3.1925426677448238e-17 0.91204751904576642 0.41008453153278329]  FollAlignAxisA=+X  BaseAlignAxisA=+Y  FollAlignAxisB=+Y  BaseAlignAxisB=+Z  BlockFunction=simmechanics.library.frames_transforms.rigid_transform
  Transform7 : sm_lib/Frames and Transforms/Rigid Transform  TranslationMethod=Cartesian  TranslationLengthUnit=mm  TranslationStandardAxis=+Z  TranslationStandardOffset=0  TranslationCartesianOffset=[13 85 85]  TranslationROffset=0  TranslationROffsetUnits=m  TranslationZOffset=0  TranslationZOffsetUnits=m  TranslationThetaOffset=0  TranslationThetaOffsetUnits=deg  RotationMethod=ArbitraryAxis  RotationAngleUnits=rad  RotationStandardAxis=+Z  RotationAngle=1.5707963267948968  RotationArbitraryAxis=[-0 -1 -0]  FollAlignAxisA=+X  BaseAlignAxisA=+Y  FollAlignAxisB=+Y  BaseAlignAxisB=+Z  BlockFunction=simmechanics.library.frames_transforms.rigid_transform
  Transform8 : sm_lib/Frames and Transforms/Rigid Transform  TranslationMethod=Cartesian  TranslationLengthUnit=mm  TranslationStandardAxis=+Z  TranslationStandardOffset=0  TranslationCartesianOffset=[-10 1 1]  TranslationROffset=0  TranslationROffsetUnits=m  TranslationZOffset=0  TranslationZOffsetUnits=m  TranslationThetaOffset=0  TranslationThetaOffsetUnits=deg  RotationMethod=ArbitraryAxis  RotationAngleUnits=rad  RotationStandardAxis=+Z  RotationAngle=2.5503618214833885  RotationArbitraryAxis=[0.67351920895470851 -0.6735192089547084 0.30453858595923028]  FollAlignAxisA=+X  BaseAlignAxisA=+Y  FollAlignAxisB=+Y  BaseAlignAxisB=+Z  BlockFunction=simmechanics.library.frames_transforms.rigid_transform
  Transform9 : sm_lib/Frames and Transforms/Rigid Transform  TranslationMethod=Cartesian  TranslationLengthUnit=mm  TranslationStandardAxis=+Z  TranslationStandardOffset=0  TranslationCartesianOffset=[-39 52.5 19]  TranslationROffset=0  TranslationROffsetUnits=m  TranslationZOffset=0  TranslationZOffsetUnits=m  TranslationThetaOffset=0  TranslationThetaOffsetUnits=deg  RotationMethod=ArbitraryAxis  RotationAngleUnits=rad  RotationStandardAxis=+Z  RotationAngle=3.1415926535897905  RotationArbitraryAxis=[-0.57504174666649199 0.81812406735821563 2.040515663386459e-15]  FollAlignAxisA=+X  BaseAlignAxisA=+Y  FollAlignAxisB=+Y  BaseAlignAxisB=+Z  BlockFunction=simmechanics.library.frames_transforms.rigid_transform
  x15060_MEAS_Capteur_deffort_1000_N_FN_9620_AA_DEFAULT_1_RIGID : Subsystem
  x15060_M_01035_Pied_porte_capteur_AA_DEFAULT_1_RIGID : Subsystem
  x15060_M_01039_Plaque_roulette_AA_DEFAULT_1_RIGID : Subsystem
  x15060_M_01063_Rondelle_entretoise_AA_DEFAULT_1_RIGID : Subsystem
  x15060_M_01063_Rondelle_entretoise_AA_DEFAULT_2_RIGID : Subsystem
  x15060_M_01063_Rondelle_entretoise_AA_DEFAULT_3_RIGID : Subsystem
  x15060_M_01063_Rondelle_entretoise_AA_DEFAULT_4_RIGID : Subsystem
  x15060_M_01063_Rondelle_entretoise_AA_DEFAULT_5_RIGID : Subsystem
  x15060_M_01069_Bride_doigt_dindexage_AA_DEFAULT_1_RIGID : Subsystem
  x15060_M_01075_Broche_M12_Modifi_e_27810_120451_1_RIGID : Subsystem
  x15060_NLM_Doigt_dindexage_acier_6_avec_contre_ecrou_M12x1_5_03 : Subsystem
  x15060_NLM_Embase_60_27801_20601_1_RIGID : Subsystem
  x15060_NLM_Roulette_pivotante_F_200_KG_95034_07532_1_RIGID : Subsystem
  x15060_NLM_Verin_a_levier_Rot_a_droite_traction_04410_35_1_RIGI : Subsystem
  x15060_Rondelle_Rondelle_Large_L_6_1_RIGID : Subsystem
  x15060_Vis_CHc_vis_CHc_M_5_X_20_1_RIGID : Subsystem
  x15060_Vis_CHc_vis_CHc_M_6_X_16_1_RIGID : Subsystem
  x15060_Vis_CHc_vis_CHc_M_8_X_12_1_RIGID : Subsystem
  x15060_Vis_CHc_vis_CHc_M_8_X_25_1_RIGID : Subsystem
  x15060_Vis_CHc_vis_CHc_M_8_X_25_2_RIGID : Subsystem
  F : PMIOPort  Port=1  Side=Right
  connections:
  Transform/RConn1 -- x15060_M_01069_Bride_doigt_dindexage_AA_DEFAULT_1_RIGID/LConn1
  Transform1/RConn1 -- x15060_Vis_CHc_vis_CHc_M_8_X_25_1_RIGID/LConn1
  Transform10/RConn1 -- x15060_M_01063_Rondelle_entretoise_AA_DEFAULT_2_RIGID/LConn1
  Transform11/RConn1 -- x15060_NLM_Verin_a_levier_Rot_a_droite_traction_04410_35_1_RIGI/LConn1
  Transform12/RConn1 -- x15060_Rondelle_Rondelle_Large_L_6_1_RIGID/LConn1
  Transform13/RConn1 -- x15060_Vis_CHc_vis_CHc_M_8_X_12_1_RIGID/LConn1
  Transform14/RConn1 -- x15060_Vis_CHc_vis_CHc_M_8_X_25_2_RIGID/LConn1
  Transform15/RConn1 -- x15060_M_01063_Rondelle_entretoise_AA_DEFAULT_5_RIGID/LConn1
  Transform16/RConn1 -- x15060_NLM_Roulette_pivotante_F_200_KG_95034_07532_1_RIGID/LConn1
  Transform17/RConn1 -- x15060_M_01063_Rondelle_entretoise_AA_DEFAULT_4_RIGID/LConn1
  Transform18/RConn1 -- x15060_MEAS_Capteur_deffort_1000_N_FN_9620_AA_DEFAULT_1_RIGID/LConn1
  Transform19/RConn1 -- x15060_M_01063_Rondelle_entretoise_AA_DEFAULT_3_RIGID/LConn1
  Transform2/RConn1 -- x15060_Vis_CHc_vis_CHc_M_6_X_16_1_RIGID/LConn1
  Transform/LConn1 -- ReferenceFrame/RConn1 -- Transform1/LConn1 -- Transform10/LConn1 -- Transform11/LConn1 -- Transform12/LConn1 -- Transform13/LConn1 -- Transform14/LConn1 -- Transform15/LConn1 -- Transform16/LConn1 -- Transform17/LConn1 -- Transform18/LConn1 -- Transform19/LConn1 -- Transform2/LConn1 -- Transform20/RConn1 -- Transform3/LConn1 -- Transform4/LConn1 -- Transform5/LConn1 -- Transform6/LConn1 -- Transform7/LConn1 -- Transform8/LConn1 -- Transform9/LConn1
  Transform20/LConn1 -- F/RConn1
  Transform3/RConn1 -- x15060_NLM_Embase_60_27801_20601_1_RIGID/LConn1
  Transform4/RConn1 -- x15060_NLM_Doigt_dindexage_acier_6_avec_contre_ecrou_M12x1_5_03/LConn1
  Transform5/RConn1 -- x15060_M_01035_Pied_porte_capteur_AA_DEFAULT_1_RIGID/LConn1
  Transform6/RConn1 -- x15060_M_01075_Broche_M12_Modifi_e_27810_120451_1_RIGID/LConn1
  Transform7/RConn1 -- x15060_M_01039_Plaque_roulette_AA_DEFAULT_1_RIGID/LConn1
  Transform8/RConn1 -- x15060_M_01063_Rondelle_entretoise_AA_DEFAULT_1_RIGID/LConn1
  Transform9/RConn1 -- x15060_Vis_CHc_vis_CHc_M_5_X_20_1_RIGID/LConn1
